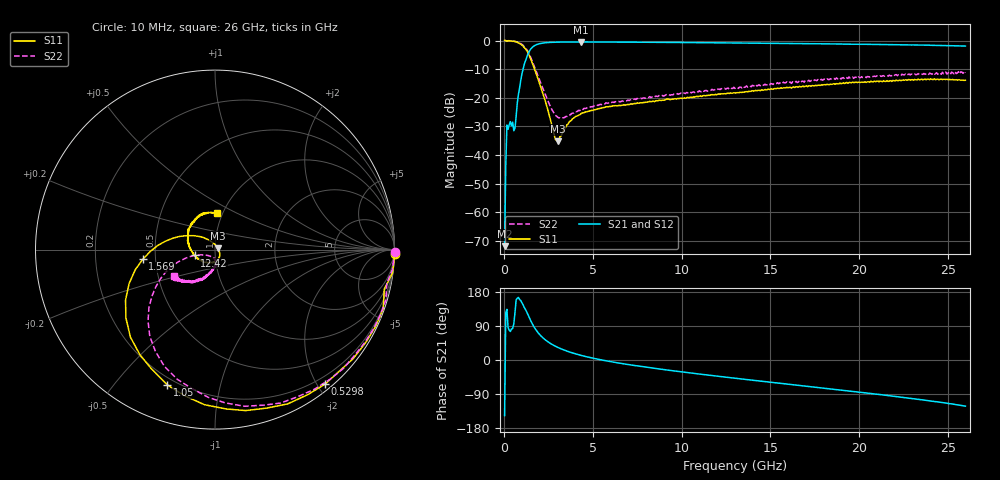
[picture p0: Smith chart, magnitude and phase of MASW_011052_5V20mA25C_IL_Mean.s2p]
! MA-COM, USA
! Part Number: MASW-011052
! Data: 29-03-2013
! Bias Condition:
!  Insertion Loss in ON stage Antenna (1) to RFin (2)
!  Forward Bias (series Diode and Shunt Diode) I = 20 mA
!  Reverse Bias Voltage V = -5V
!  Temp: 25C
!  VAR RecID: Mean
# HZ S DB R 50
! F n11x n11y n21x n21y n12x n12y n22x n22y
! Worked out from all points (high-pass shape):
!   401 points, 10 MHz to 26 GHz, reference 50 ohm
!   highest |S21| = -0.50 dB at 4.298 GHz (marker M1); lowest = -71.8 dB at 10 MHz (marker M2)
!   |S21| within 3 dB of the highest: 1.427 GHz to end of sweep
!   lowest |S11| = -35.2 dB at 2.999 GHz (marker M3), VSWR 1.04, Z = 51.6 + j0.8 ohm
!   |S11| at or under -10 dB: 1.7 GHz to end of sweep
!   |S22| runs from -27.2 to 0.0 dB; largest |S21 - S12| = 0.013
!   S11 on the Smith chart (normalised r, x): 10 MHz: -12, -89; 529.8 MHz: 0.09, -2.11; 1.05 GHz: 0.17, -0.69; 1.569 GHz: 0.42, -0.06; 12.42 GHz: 0.79, -0.05; 26 GHz: 0.94, +0.40
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1e7  0.03 -1.3  -71.83 -146.6  -80.34 -128.5  0.00 -0.8
2.0493e8  -0.06 -19.3  -31.02 85.7  -31.06 85.7  -0.06 -16.2
2.699e8  -0.07 -25.4  -29.40 78.5  -29.43 78.6  -0.09 -21.4
5.298e8  -0.28 -50.7  -31.50 95.7  -31.53 95.9  -0.22 -42.9
6.5975e8  -0.44 -64.8  -26.52 159.0  -26.54 159.2  -0.40 -54.6
7.897e8  -0.79 -79.2  -18.84 165.2  -18.86 165.4  -0.63 -66.8
1.0496e9  -1.95 -109.4  -10.09 145.6  -10.10 145.8  -1.67 -92.5
1.3095e9  -4.07 -142.4  -4.95 121.3  -4.95 121.5  -3.65 -120.3
1.5694e9  -7.82 -172.3  -2.39 95.6  -2.39 95.7  -7.20 -143.6
1.8293e9  -12.26 165.0  -1.38 76.2  -1.37 76.3  -11.33 -157.7
2.2192e9  -19.45 137.8  -0.84 56.5  -0.83 56.6  -17.49 -164.2
2.8039e9  -32.85 75.5  -0.60 38.0  -0.60 38.0  -25.38 -142.9
2.9989e9  -35.24 26.6  -0.56 33.5  -0.57 33.5  -26.77 -129.0
3.6486e9  -28.46 -44.1  -0.51 21.5  -0.52 21.5  -25.88 -95.7
4.2984e9  -25.71 -65.9  -0.50 12.5  -0.51 12.6  -24.15 -84.6
4.3633e9  -25.29 -65.8  -0.50 11.7  -0.51 11.8  -23.86 -86.8
8.7167e9  -20.87 -129.1  -0.63 -23.7  -0.64 -23.5  -19.23 -93.7
1.242e10  -18.54 -164.2  -0.80 -45.0  -0.82 -44.8  -16.70 -105.4
1.3005e10  -18.31 -167.4  -0.84 -48.0  -0.83 -47.9  -16.73 -107.6
1.7358e10  -15.73 158.9  -1.10 -70.9  -1.14 -70.7  -13.83 -121.2
2.1712e10  -14.15 127.8  -1.40 -94.3  -1.41 -94.0  -12.09 -133.6
2.6e10  -13.88 86.6  -1.93 -121.7  -1.98 -121.2  -11.28 -147.7
